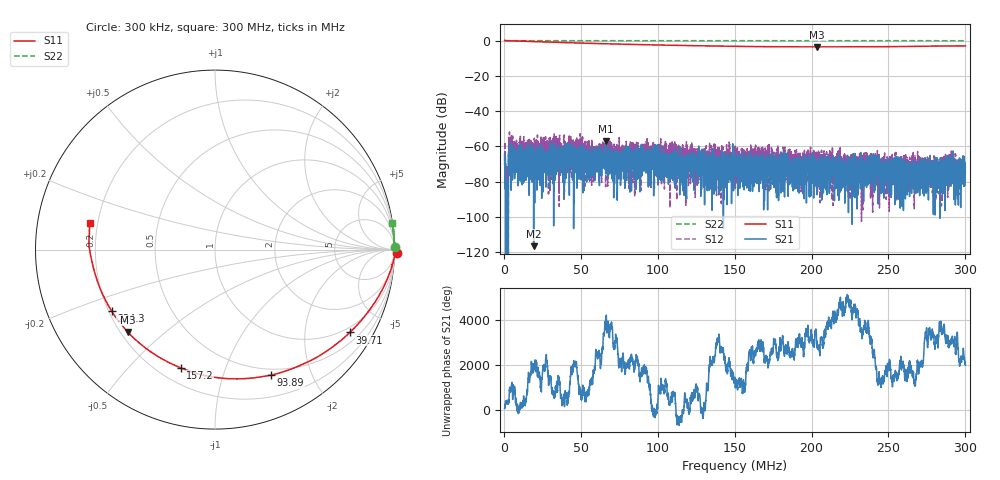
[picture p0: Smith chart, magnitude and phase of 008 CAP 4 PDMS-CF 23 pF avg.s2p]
!  26/06/2025  15:37:53
! Ref Plane: 0.000 mm
# MHZ S MA R  50
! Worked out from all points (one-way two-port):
!   4001 points, 300 kHz to 300 MHz, reference 50 ohm
!   highest |S21| = -57.12 dB at 66.01 MHz (marker M1); lowest = -116.6 dB at 19.18 MHz (marker M2)
!   lowest |S11| = -3.5 dB at 203.7 MHz (marker M3), VSWR 5.02, Z = 11.5 - j19 ohm
!   |S11| at or under -10 dB: nowhere
!   |S22| runs from 0.0 to 0.1 dB; largest |S21 - S12| = 0.0032
!   S11 on the Smith chart (normalised r, x): 300 kHz: -55, -66; 39.71 MHz: 0.81, -3.36; 93.89 MHz: 0.43, -1.45; 157.2 MHz: 0.29, -0.71; 224.3 MHz: 0.21, -0.26; 300 MHz: 0.17, +0.10
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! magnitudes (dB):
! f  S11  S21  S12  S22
! 300 kHz  0.1  -67.5  -70.5  0.0
! 1.948 MHz  0.0  -  -73.2  0.0
! 4.346 MHz  -0.1  -64.8  -59.8  0.0
! 8.467 MHz  -0.2  -64.6  -66.1  0.0
! 19.18 MHz  -0.5  -116.6  -62.8  0.0
! 39.71 MHz  -1.1  -67.6  -57.3  0.0
! 50.28 MHz  -1.4  -68.0  -67.4  0.0
! 66.01 MHz  -1.7  -57.1  -82.9  0.0
! 85.42 MHz  -2.2  -69.4  -72.9  0.0
! 93.89 MHz  -2.3  -69.3  -67.8  0.0
! 100.3 MHz  -2.4  -73.3  -71.4  0.0
! 150.2 MHz  -3.2  -72.7  -62.5  0.0
! 157.2 MHz  -3.3  -68.8  -70.2  0.0
! 172.9 MHz  -3.4  -69.4  -66.2  0.0
! 177.1 MHz  -3.4  -86.4  -70.8  0.0
! 183.1 MHz  -3.5  -63.9  -67.4  0.0
! 200.1 MHz  -3.5  -67.2  -64.4  0.0
! 203.7 MHz  -3.5  -68.2  -67.8  0.0
! 224.3 MHz  -3.5  -79.3  -73.6  0.0
! 241.6 MHz  -3.4  -70.0  -83.0  0.0
! 250.1 MHz  -3.4  -75.5  -69.0  0.0
! 300 MHz  -2.9  -71.9  -72.4  0.0
